FUNCTION_BLOCK FB_SDORead
VAR_IN_OUT 
	SDORead		:AccessSDO;		(* rising edge starts reading to the CoE Object *)
END_VAR
VAR_INPUT
	nSlaveAddr 	:UINT; 			(* Port Number of EtherCAT Slave *)
	sNetId     	:T_AmsNetId;	(* NetId of EtherCAT Master *)
END_VAR
VAR_OUTPUT
	bError		: BOOL;
    nErrId		: UDINT;
END_VAR
VAR
	fbSdoRead  	:FB_EcCoESdoRead;
END_VAR

fbSdoRead(		sNetId:= sNetId,
				nSlaveAddr :=nSlaveAddr,
				nIndex:=SDORead.nIndex, 
				nSubIndex :=SDORead.nSubIndex, 
				pDstBuf:= ADR(SDORead.nValue), 
				cbBufLen:=SIZEOF(SDORead.nValue),
				bExecute:=SDORead.bExecute);
				
IF NOT fbSdoRead.bBusy THEN
    SDORead.bExecute := FALSE;
    IF NOT fbSdoRead.bError THEN 
        (* read successful *)
        bError := FALSE;
        nErrId := 0;
    ELSE 
        (* read failed *)
        bError := fbSdoRead.bError;
        nErrId := fbSdoRead.nErrId;
    END_IF
    fbSdoRead(bExecute := FALSE);
END_IF

END_FUNCTION_BLOCK
